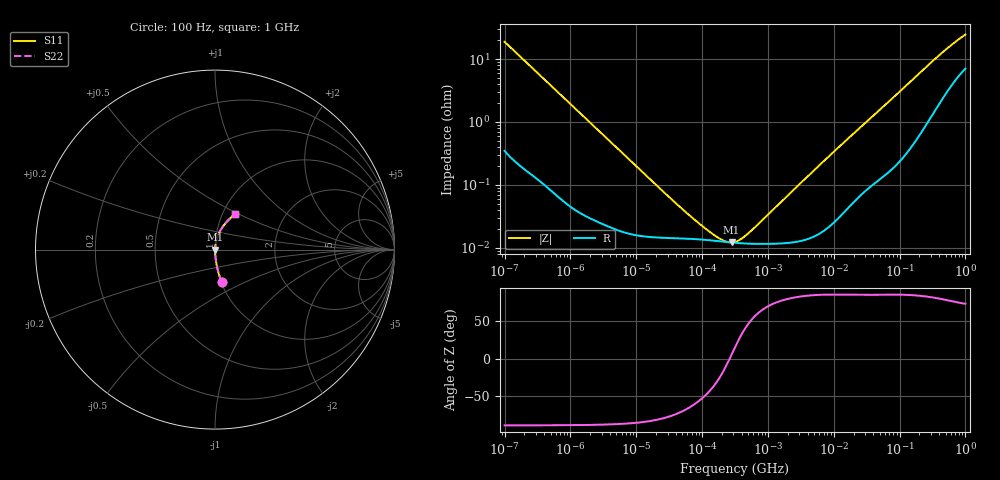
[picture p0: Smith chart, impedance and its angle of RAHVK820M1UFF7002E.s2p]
! RAHVK820M1UFF7002E  S-PARAMETER MODEL  (AEC-Q200 qualified)
! Model Generated by ELNA Corporation (http://www.ty-top.com)
! Version 1.0
! ELNA Control No. 201214
! Copyright (c) 2020 ELNA CO.,LTD. All Rights Reserved.
! Products Name : CONDUCTIVE POLYMER HYBRID ALUMINUM ELECTROLYTIC CAPACITORS
! Characteristics :
!  Capacitance  :  82uF  ,  Rated voltage  :  50V
!  Operating Temp. Range  :  -55 to +125 degC  ,  Endurance  :  4000hr at 125 degC
!  Dimension D  :  10mm  ,  Dimension L  :  8.7mm
! Frequency Range : 100Hz - 1GHz
! External Node Assignments :
!  1  o---| |---o  2
# MHz S RI R 50
!Freq[MHz].  S11 Real  S11 Imag  S21 Real  S21 Imag  S12 Real  S12 Imag  S22 Real  S22 Imag
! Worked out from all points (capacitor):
!   401 points, 100 Hz to 1 GHz, reference 50 ohm
!   read as one part in series: C = 84 uF near 108 Hz
!   lowest |Z| = 12.1 mohm at 280.2 kHz (marker M1)
!   series resonance near 262 kHz, so ESL is about 4.4 nH
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0.0001  0.0376 -0.1814  0.9624 0.1814  0.9624 0.1814  0.0376 -0.1814
0.000113  0.0301 -0.1622  0.9699 0.1622  0.9699 0.1622  0.0301 -0.1622
0.000183  0.0125 -0.1022  0.9875 0.1022  0.9875 0.1022  0.0125 -0.1022
0.000309  0.00503 -0.0614  0.995 0.0614  0.995 0.0614  0.00503 -0.0614
0.000613  0.00166 -0.0313  0.9983 0.0313  0.9983 0.0313  0.00166 -0.0313
0.001488  0.000513 -0.013  0.9995 0.013  0.9995 0.013  0.000513 -0.013
0.022131  0.000145 -0.000891  0.9999 0.000891  0.9999 0.000891  0.000145 -0.000891
0.060604  0.000139 -0.000316  0.9999 0.000316  0.9999 0.000316  0.000139 -0.000316
0.130317  0.000131 -0.000122  0.9999 0.000122  0.9999 0.000122  0.000131 -0.000122
0.203002  0.000125 -4.3e-05  0.9999 4.3e-05  0.9999 4.3e-05  0.000125 -4.3e-05
0.238506  0.000122 -1.59e-05  0.9999 1.59e-05  0.9999 1.59e-05  0.000122 -1.59e-05
0.280221  0.00012 1.15e-05  0.9999 -1.15e-05  0.9999 -1.15e-05  0.00012 1.15e-05
0.316228  0.000119 3.26e-05  0.9999 -3.26e-05  0.9999 -3.26e-05  0.000119 3.26e-05
0.402717  0.000117 7.71e-05  0.9999 -7.71e-05  0.9999 -7.71e-05  0.000117 7.71e-05
0.533949  0.000116 0.000136  0.9999 -0.000136  0.9999 -0.000136  0.000116 0.000136
4.704354  0.000148 0.00159  0.9999 -0.00159  0.9999 -0.00159  0.000148 0.00159
13.96368  0.000376 0.00463  0.9996 -0.00463  0.9996 -0.00463  0.000376 0.00463
69.9842  0.00208 0.0214  0.9979 -0.0214  0.9979 -0.0214  0.00208 0.0214
176.8072  0.00778 0.0522  0.9922 -0.0522  0.9922 -0.0522  0.00778 0.0522
380.1894  0.0286 0.1041  0.9714 -0.1041  0.9714 -0.1041  0.0286 0.1041
668.3439  0.0677 0.1573  0.9323 -0.1573  0.9323 -0.1573  0.0677 0.1573
1000  0.1098 0.1974  0.8902 -0.1974  0.8902 -0.1974  0.1098 0.1974
